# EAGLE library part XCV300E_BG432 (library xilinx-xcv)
xcv300e_bg432 edit this description Auto generated by make-symbol-device-package-bsdl.ulp Rev. 26 Source: xcv300e_bg432.bsd
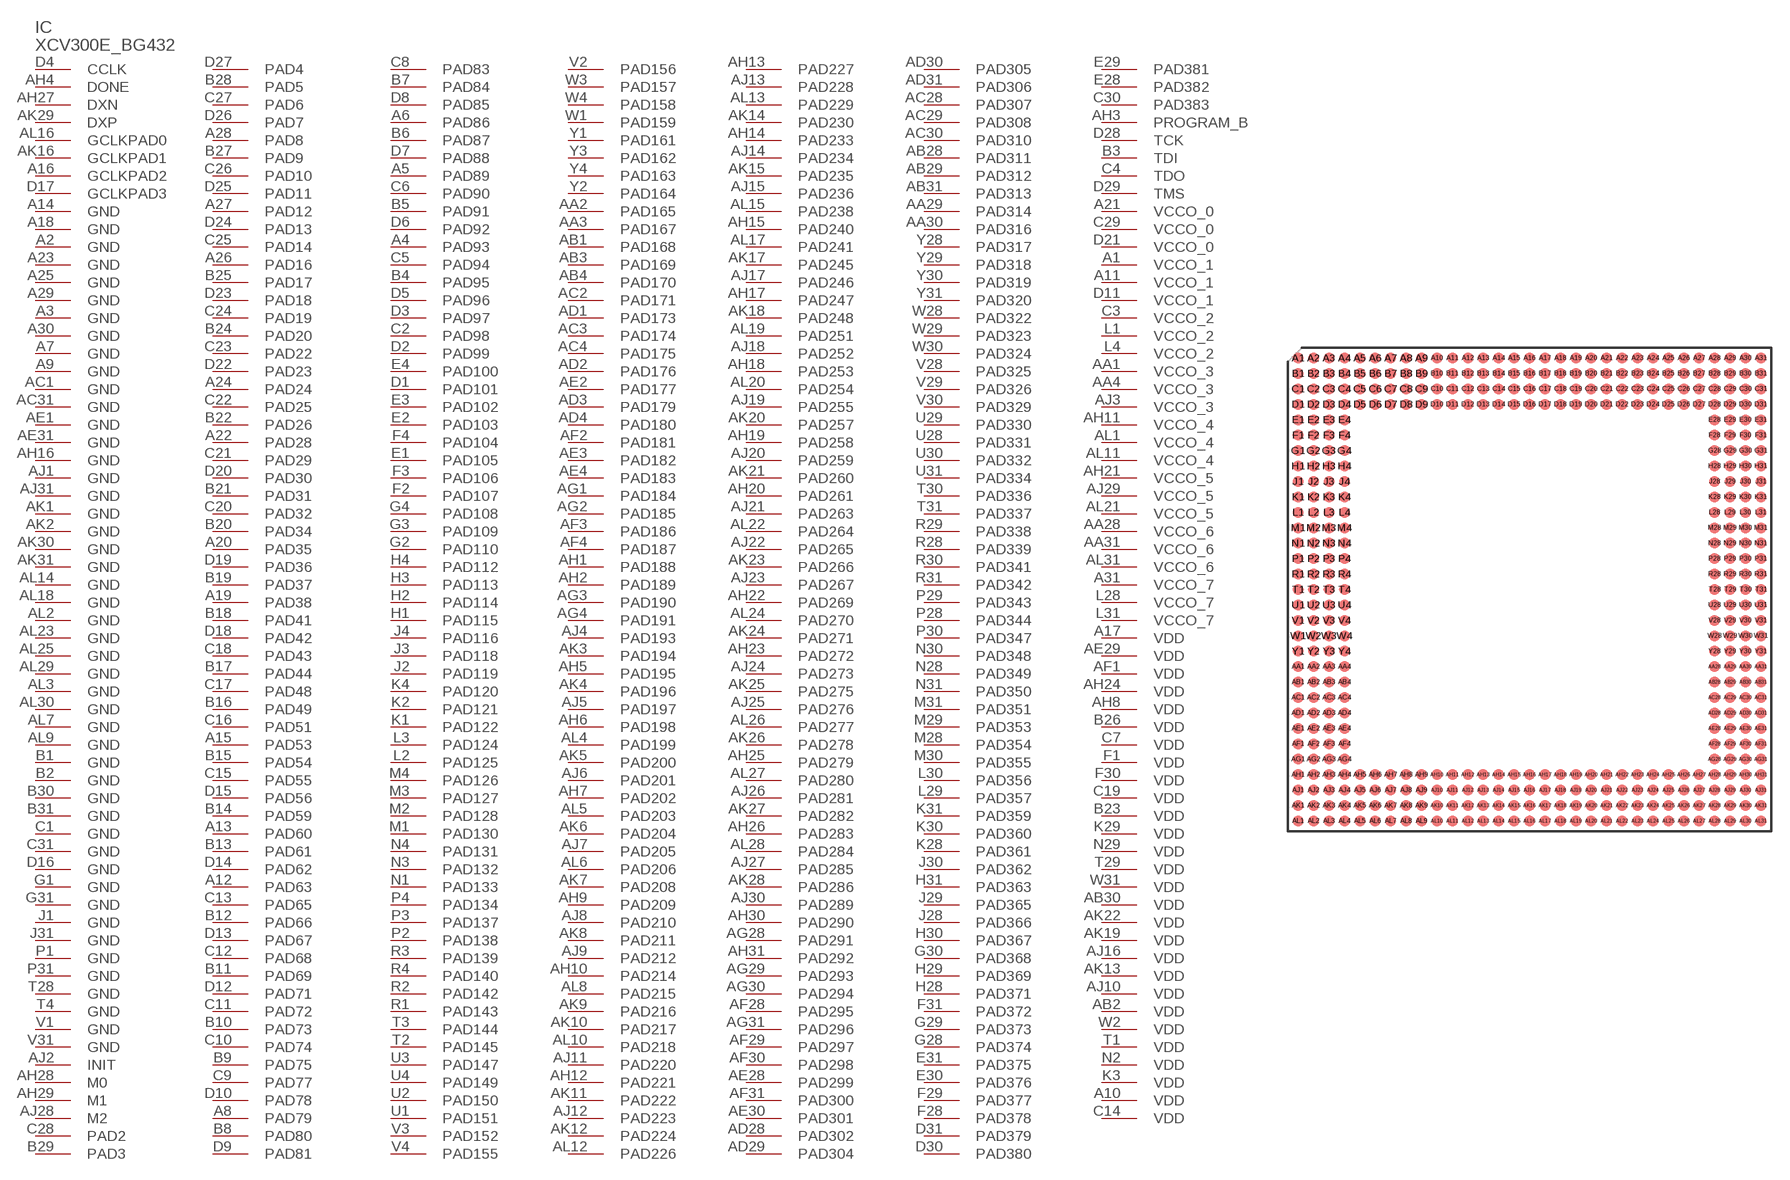
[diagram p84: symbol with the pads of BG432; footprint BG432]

Designator prefix IC

## XCV300E_BG432 (OC_FARNELL: unknown; OC_NEWARK: unknown)  [BG432]
A1  VCCO_1  pwr
A2  GND  pwr
A3  GND  pwr
A4  PAD93
A5  PAD89
A6  PAD86
A7  GND  pwr
A8  PAD79
A9  GND  pwr
A10  VDD  pwr
A11  VCCO_1  pwr
A12  PAD63
A13  PAD60
A14  GND  pwr
A15  PAD53
A16  GCLKPAD2  in
A17  VDD  pwr
A18  GND  pwr
A19  PAD38
A20  PAD35
A21  VCCO_0  pwr
A22  PAD28
A23  GND  pwr
A24  PAD24
A25  GND  pwr
A26  PAD16
A27  PAD12
A28  PAD8
A29  GND  pwr
A30  GND  pwr
A31  VCCO_7  pwr
AA1  VCCO_3  pwr
AA2  PAD165
AA3  PAD167
AA4  VCCO_3  pwr
AA28  VCCO_6  pwr
AA29  PAD314
AA30  PAD316
AA31  VCCO_6  pwr
AB1  PAD168
AB2  VDD  pwr
AB3  PAD169
AB4  PAD170
AB28  PAD311
AB29  PAD312
AB30  VDD  pwr
AB31  PAD313
AC1  GND  pwr
AC2  PAD171
AC3  PAD174
AC4  PAD175
AC28  PAD307
AC29  PAD308
AC30  PAD310
AC31  GND  pwr
AD1  PAD173
AD2  PAD176
AD3  PAD179
AD4  PAD180
AD28  PAD302
AD29  PAD304
AD30  PAD305
AD31  PAD306
AE1  GND  pwr
AE2  PAD177
AE3  PAD182
AE4  PAD183
AE28  PAD299
AE29  VDD  pwr
AE30  PAD301
AE31  GND  pwr
AF1  VDD  pwr
AF2  PAD181
AF3  PAD186
AF4  PAD187
AF28  PAD295
AF29  PAD297
AF30  PAD298
AF31  PAD300
AG1  PAD184
AG2  PAD185
AG3  PAD190
AG4  PAD191
AG28  PAD291
AG29  PAD293
AG30  PAD294
AG31  PAD296
AH1  PAD188
AH2  PAD189
AH3  PROGRAM_B  in
AH4  DONE
AH5  PAD195
AH6  PAD198
AH7  PAD202
AH8  VDD  pwr
AH9  PAD209
AH10  PAD214
AH11  VCCO_4  pwr
AH12  PAD221
AH13  PAD227
AH14  PAD233
AH15  PAD240
AH16  GND  pwr
AH17  PAD247
AH18  PAD253
AH19  PAD258
AH20  PAD261
AH21  VCCO_5  pwr
AH22  PAD269
AH23  PAD272
AH24  VDD  pwr
AH25  PAD279
AH26  PAD283
AH27  DXN  pas
AH28  M0  in
AH29  M1  in
AH30  PAD290
AH31  PAD292
AJ1  GND  pwr
AJ2  INIT
AJ3  VCCO_3  pwr
AJ4  PAD193
AJ5  PAD197
AJ6  PAD201
AJ7  PAD205
AJ8  PAD210
AJ9  PAD212
AJ10  VDD  pwr
AJ11  PAD220
AJ12  PAD223
AJ13  PAD228
AJ14  PAD234
AJ15  PAD236
AJ16  VDD  pwr
AJ17  PAD246
AJ18  PAD252
AJ19  PAD255
AJ20  PAD259
AJ21  PAD263
AJ22  PAD265
AJ23  PAD267
AJ24  PAD273
AJ25  PAD276
AJ26  PAD281
AJ27  PAD285
AJ28  M2  in
AJ29  VCCO_5  pwr
AJ30  PAD289
AJ31  GND  pwr
AK1  GND  pwr
AK2  GND  pwr
AK3  PAD194
AK4  PAD196
AK5  PAD200
AK6  PAD204
AK7  PAD208
AK8  PAD211
AK9  PAD216
AK10  PAD217
AK11  PAD222
AK12  PAD224
AK13  VDD  pwr
AK14  PAD230
AK15  PAD235
AK16  GCLKPAD1  in
AK17  PAD245
AK18  PAD248
AK19  VDD  pwr
AK20  PAD257
AK21  PAD260
AK22  VDD  pwr
AK23  PAD266
AK24  PAD271
AK25  PAD275
AK26  PAD278
AK27  PAD282
AK28  PAD286
AK29  DXP  pas
AK30  GND  pwr
AK31  GND  pwr
AL1  VCCO_4  pwr
AL2  GND  pwr
AL3  GND  pwr
AL4  PAD199
AL5  PAD203
AL6  PAD206
AL7  GND  pwr
AL8  PAD215
AL9  GND  pwr
AL10  PAD218
AL11  VCCO_4  pwr
AL12  PAD226
AL13  PAD229
AL14  GND  pwr
AL15  PAD238
AL16  GCLKPAD0  in
AL17  PAD241
AL18  GND  pwr
AL19  PAD251
AL20  PAD254
AL21  VCCO_5  pwr
AL22  PAD264
AL23  GND  pwr
AL24  PAD270
AL25  GND  pwr
AL26  PAD277
AL27  PAD280
AL28  PAD284
AL29  GND  pwr
AL30  GND  pwr
AL31  VCCO_6  pwr
B1  GND  pwr
B2  GND  pwr
B3  TDI  in
B4  PAD95
B5  PAD91
B6  PAD87
B7  PAD84
B8  PAD80
B9  PAD75
B10  PAD73
B11  PAD69
B12  PAD66
B13  PAD61
B14  PAD59
B15  PAD54
B16  PAD49
B17  PAD44
B18  PAD41
B19  PAD37
B20  PAD34
B21  PAD31
B22  PAD26
B23  VDD  pwr
B24  PAD20
B25  PAD17
B26  VDD  pwr
B27  PAD9
B28  PAD5
B29  PAD3
B30  GND  pwr
B31  GND  pwr
C1  GND  pwr
C2  PAD98
C3  VCCO_2  pwr
C4  TDO  out
C5  PAD94
C6  PAD90
C7  VDD  pwr
C8  PAD83
C9  PAD77
C10  PAD74
C11  PAD72
C12  PAD68
C13  PAD65
C14  VDD  pwr
C15  PAD55
C16  PAD51
C17  PAD48
C18  PAD43
C19  VDD  pwr
C20  PAD32
C21  PAD29
C22  PAD25
C23  PAD22
C24  PAD19
C25  PAD14
C26  PAD10
C27  PAD6
C28  PAD2
C29  VCCO_0  pwr
C30  PAD383
C31  GND  pwr
D1  PAD101
D2  PAD99
D3  PAD97
D4  CCLK
D5  PAD96
D6  PAD92
D7  PAD88
D8  PAD85
D9  PAD81
D10  PAD78
D11  VCCO_1  pwr
D12  PAD71
D13  PAD67
D14  PAD62
D15  PAD56
D16  GND  pwr
D17  GCLKPAD3  in
D18  PAD42
D19  PAD36
D20  PAD30
D21  VCCO_0  pwr
D22  PAD23
D23  PAD18
D24  PAD13
D25  PAD11
D26  PAD7
D27  PAD4
D28  TCK  in
D29  TMS  in
D30  PAD380
D31  PAD379
E1  PAD105
E2  PAD103
E3  PAD102
E4  PAD100
E28  PAD382
E29  PAD381
E30  PAD376
E31  PAD375
F1  VDD  pwr
F2  PAD107
F3  PAD106
F4  PAD104
F28  PAD378
F29  PAD377
F30  VDD  pwr
F31  PAD372
G1  GND  pwr
G2  PAD110
G3  PAD109
G4  PAD108
G28  PAD374
G29  PAD373
G30  PAD368
G31  GND  pwr
H1  PAD115
H2  PAD114
H3  PAD113
H4  PAD112
H28  PAD371
H29  PAD369
H30  PAD367
H31  PAD363
J1  GND  pwr
J2  PAD119
J3  PAD118
J4  PAD116
J28  PAD366
J29  PAD365
J30  PAD362
J31  GND  pwr
K1  PAD122
K2  PAD121
K3  VDD  pwr
K4  PAD120
K28  PAD361
K29  VDD  pwr
K30  PAD360
K31  PAD359
L1  VCCO_2  pwr
L2  PAD125
L3  PAD124
L4  VCCO_2  pwr
L28  VCCO_7  pwr
L29  PAD357
L30  PAD356
L31  VCCO_7  pwr
M1  PAD130
M2  PAD128
M3  PAD127
M4  PAD126
M28  PAD354
M29  PAD353
M30  PAD355
M31  PAD351
N1  PAD133
N2  VDD  pwr
N3  PAD132
N4  PAD131
N28  PAD349
N29  VDD  pwr
N30  PAD348
N31  PAD350
P1  GND  pwr
P2  PAD138
P3  PAD137
P4  PAD134
P28  PAD344
P29  PAD343
P30  PAD347
P31  GND  pwr
R1  PAD143
R2  PAD142
R3  PAD139
R4  PAD140
R28  PAD339
R29  PAD338
R30  PAD341
R31  PAD342
T1  VDD  pwr
T2  PAD145
T3  PAD144
T4  GND  pwr
T28  GND  pwr
T29  VDD  pwr
T30  PAD336
T31  PAD337
U1  PAD151
U2  PAD150
U3  PAD147
U4  PAD149
U28  PAD331
U29  PAD330
U30  PAD332
U31  PAD334
V1  GND  pwr
V2  PAD156
V3  PAD152
V4  PAD155
V28  PAD325
V29  PAD326
V30  PAD329
V31  GND  pwr
W1  PAD159
W2  VDD  pwr
W3  PAD157
W4  PAD158
W28  PAD322
W29  PAD323
W30  PAD324
W31  VDD  pwr
Y1  PAD161
Y2  PAD164
Y3  PAD162
Y4  PAD163
Y28  PAD317
Y29  PAD318
Y30  PAD319
Y31  PAD320

## Footprint BG432 (pad centres in mm)
xcv300_bg432 edit this description Auto generated by make-symbol-device-package-bsdl.ulp Rev. 26 Source: xcv300_bg432.bsd
smd 0.9 x 0.9: A1 -19.05,19.05; A2 -17.78,19.05; A3 -16.51,19.05; A4 -15.24,19.05; A5 -13.97,19.05; A6 -12.7,19.05; A7 -11.43,19.05; A8 -10.16,19.05; A9 -8.89,19.05; A10 -7.62,19.05; A11 -6.35,19.05; A12 -5.08,19.05; A13 -3.81,19.05; A14 -2.54,19.05; A15 -1.27,19.05; A16 0,19.05; A17 1.27,19.05; A18 2.54,19.05; A19 3.81,19.05; A20 5.08,19.05; A21 6.35,19.05; A22 7.62,19.05; A23 8.89,19.05; A24 10.16,19.05; A25 11.43,19.05; A26 12.7,19.05; A27 13.97,19.05; A28 15.24,19.05; A29 16.51,19.05; A30 17.78,19.05; A31 19.05,19.05; AA1 -19.05,-6.35; AA2 -17.78,-6.35; AA3 -16.51,-6.35; AA4 -15.24,-6.35; AA28 15.24,-6.35; AA29 16.51,-6.35; AA30 17.78,-6.35; AA31 19.05,-6.35; AB1 -19.05,-7.62; AB2 -17.78,-7.62; AB3 -16.51,-7.62; AB4 -15.24,-7.62; AB28 15.24,-7.62; AB29 16.51,-7.62; AB30 17.78,-7.62; AB31 19.05,-7.62; AC1 -19.05,-8.89; AC2 -17.78,-8.89; AC3 -16.51,-8.89; AC4 -15.24,-8.89; AC28 15.24,-8.89; AC29 16.51,-8.89; AC30 17.78,-8.89; AC31 19.05,-8.89; AD1 -19.05,-10.16; AD2 -17.78,-10.16; AD3 -16.51,-10.16; AD4 -15.24,-10.16; AD28 15.24,-10.16; AD29 16.51,-10.16; AD30 17.78,-10.16; AD31 19.05,-10.16; AE1 -19.05,-11.43; AE2 -17.78,-11.43; AE3 -16.51,-11.43; AE4 -15.24,-11.43; AE28 15.24,-11.43; AE29 16.51,-11.43; AE30 17.78,-11.43; AE31 19.05,-11.43; AF1 -19.05,-12.7; AF2 -17.78,-12.7; AF3 -16.51,-12.7; AF4 -15.24,-12.7; AF28 15.24,-12.7; AF29 16.51,-12.7; AF30 17.78,-12.7; AF31 19.05,-12.7; AG1 -19.05,-13.97; AG2 -17.78,-13.97; AG3 -16.51,-13.97; AG4 -15.24,-13.97; AG28 15.24,-13.97; AG29 16.51,-13.97; AG30 17.78,-13.97; AG31 19.05,-13.97; AH1 -19.05,-15.24; AH2 -17.78,-15.24; AH3 -16.51,-15.24; AH4 -15.24,-15.24; AH5 -13.97,-15.24; AH6 -12.7,-15.24; AH7 -11.43,-15.24; AH8 -10.16,-15.24; AH9 -8.89,-15.24; AH10 -7.62,-15.24; AH11 -6.35,-15.24; AH12 -5.08,-15.24; AH13 -3.81,-15.24; AH14 -2.54,-15.24; AH15 -1.27,-15.24; AH16 0,-15.24; AH17 1.27,-15.24; AH18 2.54,-15.24; AH19 3.81,-15.24; AH20 5.08,-15.24; AH21 6.35,-15.24; AH22 7.62,-15.24; AH23 8.89,-15.24; AH24 10.16,-15.24; AH25 11.43,-15.24; AH26 12.7,-15.24; AH27 13.97,-15.24; AH28 15.24,-15.24; AH29 16.51,-15.24; AH30 17.78,-15.24; AH31 19.05,-15.24; AJ1 -19.05,-16.51; AJ2 -17.78,-16.51; AJ3 -16.51,-16.51; AJ4 -15.24,-16.51; AJ5 -13.97,-16.51; AJ6 -12.7,-16.51; AJ7 -11.43,-16.51; AJ8 -10.16,-16.51; AJ9 -8.89,-16.51; AJ10 -7.62,-16.51; AJ11 -6.35,-16.51; AJ12 -5.08,-16.51; AJ13 -3.81,-16.51; AJ14 -2.54,-16.51; AJ15 -1.27,-16.51; AJ16 0,-16.51; AJ17 1.27,-16.51; AJ18 2.54,-16.51; AJ19 3.81,-16.51; AJ20 5.08,-16.51; AJ21 6.35,-16.51; AJ22 7.62,-16.51; AJ23 8.89,-16.51; AJ24 10.16,-16.51; AJ25 11.43,-16.51; AJ26 12.7,-16.51; AJ27 13.97,-16.51; AJ28 15.24,-16.51; AJ29 16.51,-16.51; AJ30 17.78,-16.51; AJ31 19.05,-16.51; AK1 -19.05,-17.78; AK2 -17.78,-17.78; AK3 -16.51,-17.78; AK4 -15.24,-17.78; AK5 -13.97,-17.78; AK6 -12.7,-17.78; AK7 -11.43,-17.78; AK8 -10.16,-17.78; AK9 -8.89,-17.78; AK10 -7.62,-17.78; AK11 -6.35,-17.78; AK12 -5.08,-17.78; AK13 -3.81,-17.78; AK14 -2.54,-17.78; AK15 -1.27,-17.78; AK16 0,-17.78; AK17 1.27,-17.78; AK18 2.54,-17.78; AK19 3.81,-17.78; AK20 5.08,-17.78; AK21 6.35,-17.78; AK22 7.62,-17.78; AK23 8.89,-17.78; AK24 10.16,-17.78; AK25 11.43,-17.78; AK26 12.7,-17.78; AK27 13.97,-17.78; AK28 15.24,-17.78; AK29 16.51,-17.78; AK30 17.78,-17.78; AK31 19.05,-17.78; AL1 -19.05,-19.05; AL2 -17.78,-19.05; AL3 -16.51,-19.05; AL4 -15.24,-19.05; AL5 -13.97,-19.05; AL6 -12.7,-19.05; AL7 -11.43,-19.05; AL8 -10.16,-19.05; AL9 -8.89,-19.05; AL10 -7.62,-19.05; AL11 -6.35,-19.05; AL12 -5.08,-19.05; AL13 -3.81,-19.05; AL14 -2.54,-19.05; AL15 -1.27,-19.05; AL16 0,-19.05; AL17 1.27,-19.05; AL18 2.54,-19.05; AL19 3.81,-19.05; AL20 5.08,-19.05; AL21 6.35,-19.05; AL22 7.62,-19.05; AL23 8.89,-19.05; AL24 10.16,-19.05; AL25 11.43,-19.05; AL26 12.7,-19.05; AL27 13.97,-19.05; AL28 15.24,-19.05; AL29 16.51,-19.05; AL30 17.78,-19.05; AL31 19.05,-19.05; B1 -19.05,17.78; B2 -17.78,17.78; B3 -16.51,17.78; B4 -15.24,17.78; B5 -13.97,17.78; B6 -12.7,17.78; B7 -11.43,17.78; B8 -10.16,17.78; B9 -8.89,17.78; B10 -7.62,17.78; B11 -6.35,17.78; B12 -5.08,17.78; B13 -3.81,17.78; B14 -2.54,17.78; B15 -1.27,17.78; B16 0,17.78; B17 1.27,17.78; B18 2.54,17.78; B19 3.81,17.78; B20 5.08,17.78; B21 6.35,17.78; B22 7.62,17.78; B23 8.89,17.78; B24 10.16,17.78; B25 11.43,17.78; B26 12.7,17.78; B27 13.97,17.78; B28 15.24,17.78; B29 16.51,17.78; B30 17.78,17.78; B31 19.05,17.78; C1 -19.05,16.51; C2 -17.78,16.51; C3 -16.51,16.51; C4 -15.24,16.51; C5 -13.97,16.51; C6 -12.7,16.51; C7 -11.43,16.51; C8 -10.16,16.51; C9 -8.89,16.51; C10 -7.62,16.51; C11 -6.35,16.51; C12 -5.08,16.51; C13 -3.81,16.51; C14 -2.54,16.51; C15 -1.27,16.51; C16 0,16.51; C17 1.27,16.51; C18 2.54,16.51; C19 3.81,16.51; C20 5.08,16.51; C21 6.35,16.51; C22 7.62,16.51; C23 8.89,16.51; C24 10.16,16.51; C25 11.43,16.51; C26 12.7,16.51; C27 13.97,16.51; C28 15.24,16.51; C29 16.51,16.51; C30 17.78,16.51; C31 19.05,16.51; D1 -19.05,15.24; D2 -17.78,15.24; D3 -16.51,15.24; D4 -15.24,15.24; D5 -13.97,15.24; D6 -12.7,15.24; D7 -11.43,15.24; D8 -10.16,15.24; D9 -8.89,15.24; D10 -7.62,15.24; D11 -6.35,15.24; D12 -5.08,15.24; D13 -3.81,15.24; D14 -2.54,15.24; D15 -1.27,15.24; D16 0,15.24; D17 1.27,15.24; D18 2.54,15.24; D19 3.81,15.24; D20 5.08,15.24; D21 6.35,15.24; D22 7.62,15.24; D23 8.89,15.24; D24 10.16,15.24; D25 11.43,15.24; D26 12.7,15.24; D27 13.97,15.24; D28 15.24,15.24; D29 16.51,15.24; D30 17.78,15.24; D31 19.05,15.24; E1 -19.05,13.97; E2 -17.78,13.97; E3 -16.51,13.97; E4 -15.24,13.97; E28 15.24,13.97; E29 16.51,13.97; E30 17.78,13.97; E31 19.05,13.97; F1 -19.05,12.7; F2 -17.78,12.7; F3 -16.51,12.7; F4 -15.24,12.7; F28 15.24,12.7; F29 16.51,12.7; F30 17.78,12.7; F31 19.05,12.7; G1 -19.05,11.43; G2 -17.78,11.43; G3 -16.51,11.43; G4 -15.24,11.43; G28 15.24,11.43; G29 16.51,11.43; G30 17.78,11.43; G31 19.05,11.43; H1 -19.05,10.16; H2 -17.78,10.16; H3 -16.51,10.16; H4 -15.24,10.16; H28 15.24,10.16; H29 16.51,10.16; H30 17.78,10.16; H31 19.05,10.16; J1 -19.05,8.89; J2 -17.78,8.89; J3 -16.51,8.89; J4 -15.24,8.89; J28 15.24,8.89; J29 16.51,8.89; J30 17.78,8.89; J31 19.05,8.89; K1 -19.05,7.62; K2 -17.78,7.62; K3 -16.51,7.62; K4 -15.24,7.62; K28 15.24,7.62; K29 16.51,7.62; K30 17.78,7.62; K31 19.05,7.62; L1 -19.05,6.35; L2 -17.78,6.35; L3 -16.51,6.35; L4 -15.24,6.35; L28 15.24,6.35; L29 16.51,6.35; L30 17.78,6.35; L31 19.05,6.35; M1 -19.05,5.08; M2 -17.78,5.08; M3 -16.51,5.08; M4 -15.24,5.08; M28 15.24,5.08; M29 16.51,5.08; M30 17.78,5.08; M31 19.05,5.08; N1 -19.05,3.81; N2 -17.78,3.81; N3 -16.51,3.81; N4 -15.24,3.81; N28 15.24,3.81; N29 16.51,3.81; N30 17.78,3.81; N31 19.05,3.81; P1 -19.05,2.54; P2 -17.78,2.54; P3 -16.51,2.54; P4 -15.24,2.54; P28 15.24,2.54; P29 16.51,2.54; P30 17.78,2.54; P31 19.05,2.54; R1 -19.05,1.27; R2 -17.78,1.27; R3 -16.51,1.27; R4 -15.24,1.27; R28 15.24,1.27; R29 16.51,1.27; R30 17.78,1.27; R31 19.05,1.27; T1 -19.05,0; T2 -17.78,0; T3 -16.51,0; T4 -15.24,0; T28 15.24,0; T29 16.51,0; T30 17.78,0; T31 19.05,0; U1 -19.05,-1.27; U2 -17.78,-1.27; U3 -16.51,-1.27; U4 -15.24,-1.27; U28 15.24,-1.27; U29 16.51,-1.27; U30 17.78,-1.27; U31 19.05,-1.27; V1 -19.05,-2.54; V2 -17.78,-2.54; V3 -16.51,-2.54; V4 -15.24,-2.54; V28 15.24,-2.54; V29 16.51,-2.54; V30 17.78,-2.54; V31 19.05,-2.54; W1 -19.05,-3.81; W2 -17.78,-3.81; W3 -16.51,-3.81; W4 -15.24,-3.81; W28 15.24,-3.81; W29 16.51,-3.81; W30 17.78,-3.81; W31 19.05,-3.81; Y1 -19.05,-5.08; Y2 -17.78,-5.08; Y3 -16.51,-5.08; Y4 -15.24,-5.08; Y28 15.24,-5.08; Y29 16.51,-5.08; Y30 17.78,-5.08; Y31 19.05,-5.08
